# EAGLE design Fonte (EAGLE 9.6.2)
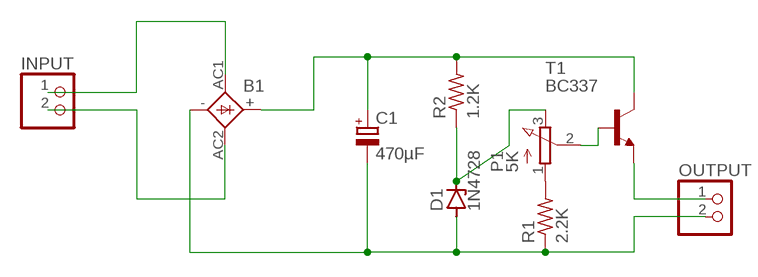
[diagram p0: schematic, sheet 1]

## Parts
B1  1KAB  [1KAB]
C1  470µF  CPOL-EUE3.5-10  [E3,5-10]
D1  1N4728  [DO41Z10]
INPUT  PINHD-1X2  [1X02]
OUTPUT  PINHD-1X2  [1X02]
P1  5K  3RP/1610N  [3RP/1610N]
R1  2.2K  R-US_0309/12  [0309/12]
R2  1.2K  R-US_0309/12  [0309/12]
T1  BC337  [TO92]

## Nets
N$1: B1.AC1 INPUT.1
N$2: B1.AC2 INPUT.2
N$3: B1.+ C1.+ R2.2 T1.3(C)
N$4: B1.- C1.- D1.A OUTPUT.2 R1.1
N$5: D1.C P1.3(E) R2.1
N$6: P1.1(A) R1.2
N$7: P1.2(S) T1.2(B)
N$8: OUTPUT.1 T1.1(E)

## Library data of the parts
B1 = rectifier:1KAB: RECTIFIER grid 5,08 x 5,08 mm
C1 = rcl:CPOL-EU: POLARIZED CAPACITOR, European symbol; SPICEPREFIX: C
D1 = diode:1N4728: Z DIODE
INPUT OUTPUT = pinhead:PINHD-1X2: PIN HEADER
P1 = pot:3RP/1610N: 16mm Potentiometer one level Source: http://www.alphapotentiometers.net/html/16mm_pot_2.html
R1 R2 = rcl:R-US_: RESISTOR, American symbol; SPICEPREFIX: R
T1 = transistor:BC337: NPN TRANSISTOR

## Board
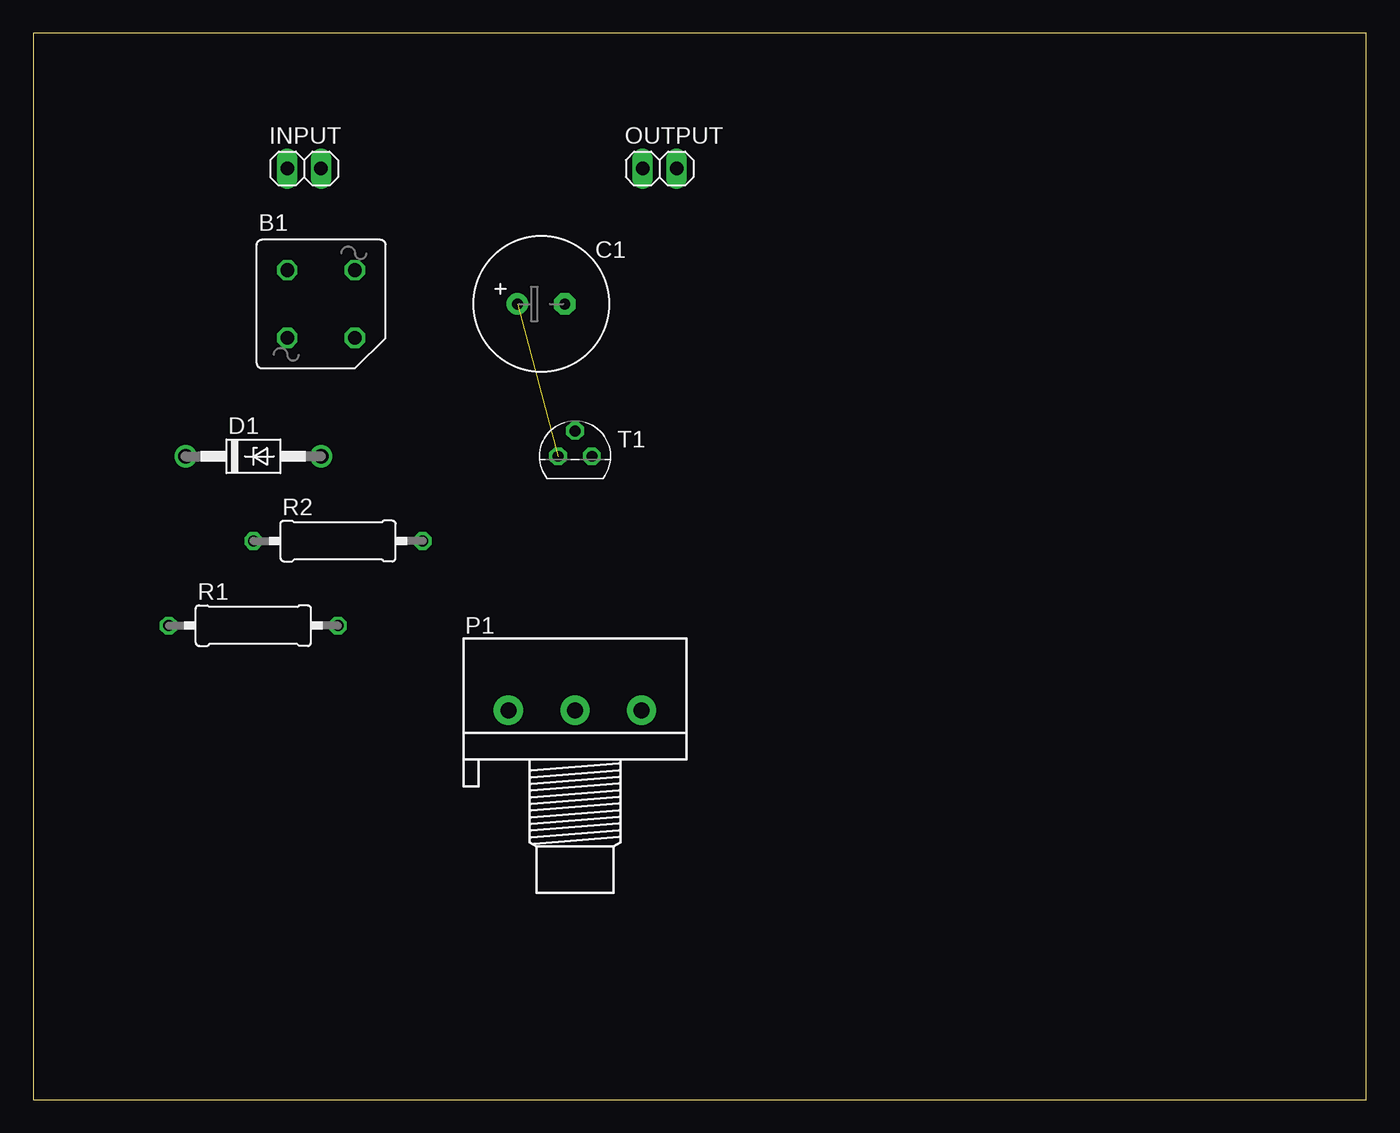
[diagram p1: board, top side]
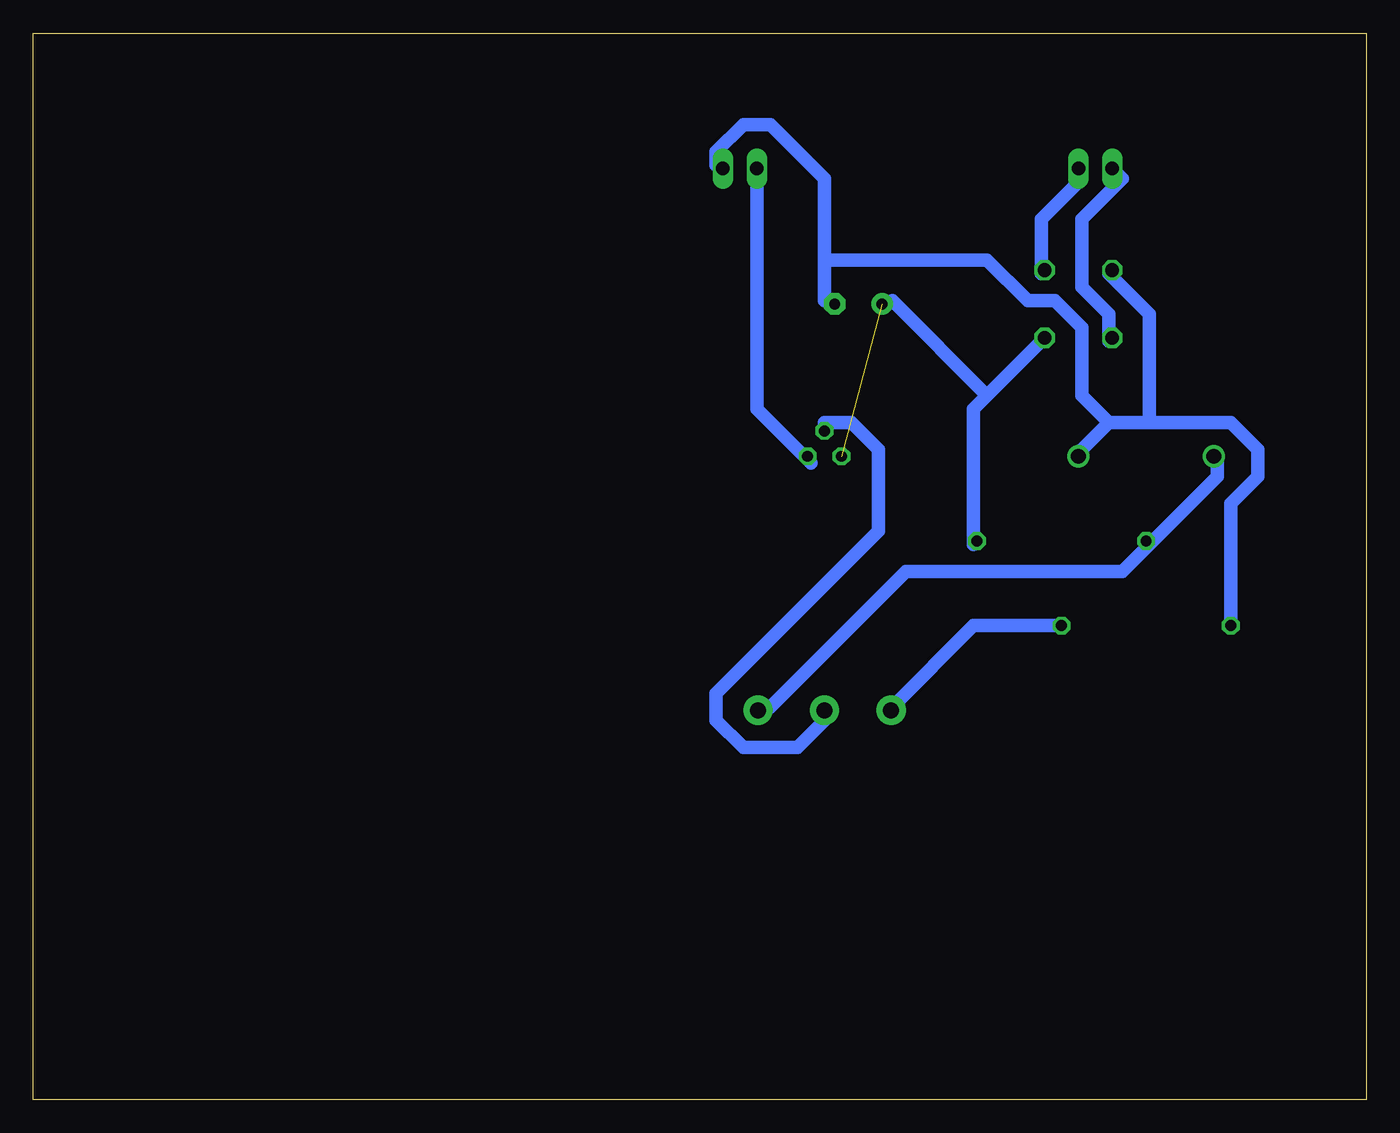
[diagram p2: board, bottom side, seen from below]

Size 100 x 80 mm. Coordinates in mm from the lower left corner, seen from the top.
Outline: 0,0 100,0 100,80 0,80 0,0
Copper layers (1*16): Top 0.035mm / dielectric 1.5mm / Bottom 0.035mm
Design rules "default *": minimum track width 40mil, minimum drill 0.35mm, track to track 40mil, track to pad 40mil, pad to pad 40mil, via to via 40mil, smd to smd 6mil, copper to edge 40mil, drill to drill 6mil, minimum pad ring 10mil, minimum via ring 8mil, stop-mask expansion 4mil, vias tented up to drill 0mil, thermal gap 10mil

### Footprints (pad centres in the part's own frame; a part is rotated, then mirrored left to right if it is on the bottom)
1KAB = drill 1.016 octagon: + 2.54,-2.54; - -2.54,2.54; AC1 -2.54,-2.54; AC2 2.54,2.54
E3,5-10 = drill 0.813 pad 1.6: + -1.778,0 | drill 0.813 pad 1.6 octagon: - 1.778,0
DO41Z10 = drill 1.118: A 5.08,0; C -5.08,0
1X02 = drill 1.016 long: 1 -1.27,0; 2 1.27,0
3RP/1610N = drill 1.2 pad 2.184: 1 -5,0; 2 0,0; 3 5,0
0309/12 = drill 0.813 octagon: 1 -6.35,0; 2 6.35,0
TO92 = drill 0.813 octagon: 1 1.27,0; 2 0,1.905; 3 -1.27,0

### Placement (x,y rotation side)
B1  21.59,59.69 0 top
C1  38.1,59.69 0 top
D1  16.51,48.26 0 top
INPUT  20.32,69.85 0 top
OUTPUT  46.99,69.85 0 top
P1  40.64,29.21 0 top
R1  16.51,35.56 0 top
R2  22.86,41.91 0 top
T1  40.64,48.26 0 top

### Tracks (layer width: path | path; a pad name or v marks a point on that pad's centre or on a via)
N$1
  Bottom 1.016: B1.AC1 19.3,56.9 19.3,58.93 21.34,60.96 21.34,66.04 18.29,69.09 INPUT.1 19.3,70.1
N$2
  Bottom 1.016: INPUT.2 21.34,69.09 24.38,66.04 24.38,61.98 B1.AC2
N$3  (1 unrouted)
  Bottom 1.016: B1.+ 28.45,52.83 | 28.45,52.83 29.46,51.82 29.46,41.66 R2.2 | 28.45,52.83 35.56,59.94 C1.+
N$4
  Bottom 1.016: 40.64,62.99 40.64,59.94 C1.- | 40.64,62.99 40.64,69.09 44.7,73.15 46.74,73.15 48.77,71.12 48.77,70.1 OUTPUT.2 | R1.1 10.16,44.7 8.13,46.74 8.13,48.77 10.16,50.8 16.26,50.8 | 19.3,50.8 16.26,50.8 | 19.3,50.8 21.34,48.77 D1.A | 16.26,50.8 16.26,58.93 19.3,61.98 B1.- | 40.64,62.99 28.45,62.99 25.4,59.94 23.37,59.94 21.34,57.91 21.34,52.83 19.3,50.8
N$5
  Bottom 1.016: 16.26,41.66 11.18,46.74 11.18,47.75 D1.C | 16.26,41.66 18.29,39.62 34.54,39.62 44.7,29.46 P1.3 | 16.26,41.66 R2.1
N$6
  Bottom 1.016: R1.2 29.46,35.56 35.56,29.46 P1.1
N$7
  Bottom 1.016: T1.2 40.64,50.8 38.61,50.8 36.58,48.77 36.58,42.67 48.77,30.48 48.77,28.45 46.74,26.42 42.67,26.42 40.64,28.45 P1.2
N$8
  Bottom 1.016: OUTPUT.1 45.72,51.82 41.66,47.75 T1.1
